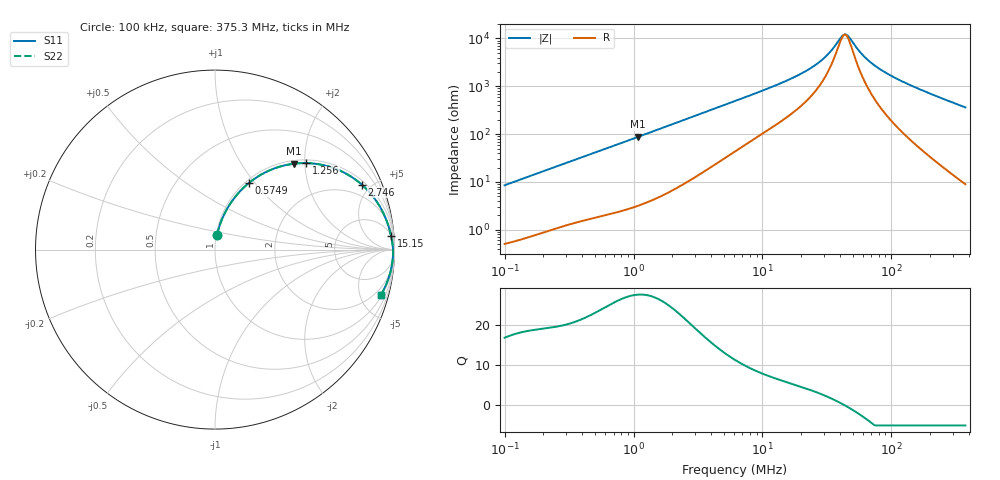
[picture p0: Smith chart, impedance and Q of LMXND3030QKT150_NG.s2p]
! LMXND3030QKT150_NG  S-PARAMETER MODEL  ( Standard Model )
! Model Generated by TAIYO YUDEN Corporation (http://www.ty-top.com)
! Version 1.0
! TAIYO YUDEN Control No. 20240226
! Copyright(c) 2024 TAIYO YUDEN CO.,LTD. All Rights Reserved.
! Product Description (link to TY-COMPAS)
! https://ds.yuden.co.jp/TYCOMPAS/or/detail?pn=LMXND3030QKT150MNG&u=M
! Products Name : Inductors
! Characteristics :
!  Inductance : 15 [uH] , SRF(min) : 23 [MHz] , DC Resistance(max) : 0.39 [Ohm]
!  Rated Current : Saturation  580 [mA] , Temp Rise  680 [mA] (40 [degC])
!  Case Size : 3.0 x 3.0 / 0.118 x 0.118 [mm/inch] , Thickness : 1.5 / 0.059 [mm/inch]
!  (Conditions: Temperature = 25 [degC] , DC Bias Current = 0 [A])
! External Node Assignments :
!  1  o---GGG---o  2
! GND o---------o GND
! Frequency Range : 0.1MHz  -  375.343504MHz  [ 402 STEP ]
# MHz S RI R 50
! Freq[MHz].  S11 Real  S11 Imag  S21 Real  S21 Imag  S12 Real  S12 Imag  S22 Real  S22 Imag
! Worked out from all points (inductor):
!   401 points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, 100 kHz to 375.3 MHz, reference 50 ohm
!   read as one part in series: L = 13.5 uH near 104.2 kHz
!   highest Q = 27.6 at 1.088 MHz (marker M1), where L = 12.8 uH
!   self-resonance near 43.27 MHz
!   S11 on the Smith chart (normalised r, x): 100 kHz: 1.01, +0.17; 574.9 kHz: 1.04, +0.94; 1.256 MHz: 1.07, +2.03; 2.746 MHz: 1.22, +4.41; 15.15 MHz: 5, +25; 375.3 MHz: 1.18, -7.24
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0.1  0.0121 0.0837  0.9879 -0.0837  0.9879 -0.0837  0.0121 0.0837
0.201292  0.0358 0.1615  0.9642 -0.1615  0.9642 -0.1615  0.0358 0.1615
0.396933  0.1072 0.2869  0.8928 -0.2869  0.8928 -0.2869  0.1072 0.2869
0.574865  0.1899 0.372  0.8101 -0.372  0.8101 -0.372  0.1899 0.372
1.087888  0.4379 0.4783  0.5621 -0.4783  0.5621 -0.4783  0.4379 0.4783
1.256426  0.5065 0.4821  0.4935 -0.4821  0.4935 -0.4821  0.5065 0.4821
1.575555  0.6129 0.4685  0.3871 -0.4685  0.3871 -0.4685  0.6129 0.4685
2.746045  0.818 0.362  0.182 -0.362  0.182 -0.362  0.818 0.362
3.977012  0.8964 0.2746  0.1036 -0.2746  0.1036 -0.2746  0.8964 0.2746
6.253894  0.9466 0.1844  0.0534 -0.1844  0.0534 -0.1844  0.9466 0.1844
15.14962  0.9815 0.0742  0.0185 -0.0742  0.0185 -0.0742  0.9815 0.0742
24.31819  0.9882 0.0376  0.0118 -0.0376  0.0118 -0.0376  0.9882 0.0376
31.12893  0.9903 0.0212  0.00974 -0.0212  0.00974 -0.0212  0.9903 0.0212
40.67552  0.9916 0.00432  0.00838 -0.00432  0.00838 -0.00432  0.9916 0.00432
44.16491  0.9919 -0.000835  0.00813 0.000835  0.00813 0.000835  0.9919 -0.000835
46.97704  0.992 -0.00473  0.008 0.00473  0.008 0.00473  0.992 -0.00473
56.53407  0.9921 -0.0166  0.00786 0.0166  0.00786 0.0166  0.9921 -0.0166
65.29242  0.992 -0.0263  0.00804 0.0263  0.00804 0.0263  0.992 -0.0263
76.97529  0.9914 -0.0381  0.00859 0.0381  0.00859 0.0381  0.9914 -0.0381
96.52685  0.9899 -0.0561  0.0101 0.0561  0.0101 0.0561  0.9899 -0.0561
171.7347  0.9795 -0.1165  0.0205 0.1165  0.0205 0.1165  0.9795 -0.1165
375.3435  0.9237 -0.2534  0.0763 0.2534  0.0763 0.2534  0.9237 -0.2534
